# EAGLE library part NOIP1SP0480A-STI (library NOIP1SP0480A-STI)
Image Sensors PYTHON480 1/3.6 BW_ CRA Source: Datasheet
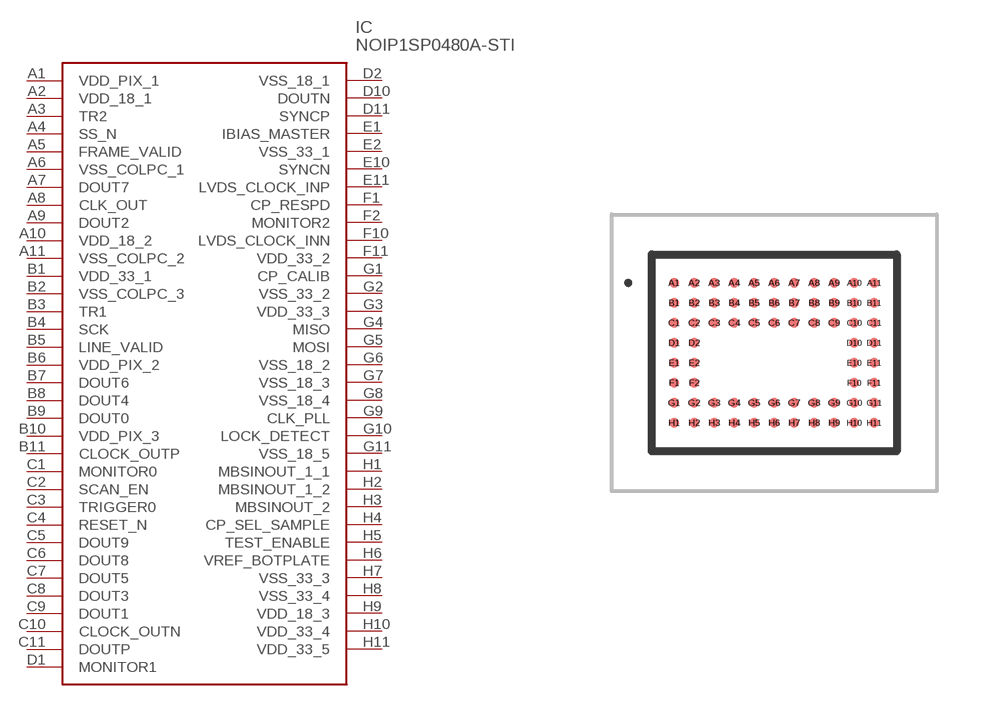
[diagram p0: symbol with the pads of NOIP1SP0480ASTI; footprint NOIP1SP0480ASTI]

Designator prefix IC

## NOIP1SP0480A-STI (Description: Image Sensors PYTHON480 1/3.6 BW_ CRA; Height: 0.75mm; Manufacturer_Name: onsemi; Manufacturer_Part_Number: NOIP1SP0480A-STI; Mouser_Part_Number: 863-NOIP1SP0480A-STI; Mouser_Price-Stock: https://www.mouser.co.uk/ProductDetail/ON-Semiconductor/NOIP1SP0480A-STI?qs=MLItCLRbWsyoZFKf%252BDS9uw%3D%3D)  [NOIP1SP0480ASTI]
A1  VDD_PIX_1
A2  VDD_18_1
A3  TR2
A4  SS_N
A5  FRAME_VALID
A6  VSS_COLPC_1
A7  DOUT7
A8  CLK_OUT
A9  DOUT2
A10  VDD_18_2
A11  VSS_COLPC_2
B1  VDD_33_1
B2  VSS_COLPC_3
B3  TR1
B4  SCK
B5  LINE_VALID
B6  VDD_PIX_2
B7  DOUT6
B8  DOUT4
B9  DOUT0
B10  VDD_PIX_3
B11  CLOCK_OUTP
C1  MONITOR0
C2  SCAN_EN
C3  TRIGGER0
C4  RESET_N
C5  DOUT9
C6  DOUT8
C7  DOUT5
C8  DOUT3
C9  DOUT1
C10  CLOCK_OUTN
C11  DOUTP
D1  MONITOR1
D2  VSS_18_1
D10  DOUTN
D11  SYNCP
E1  IBIAS_MASTER
E2  VSS_33_1
E10  SYNCN
E11  LVDS_CLOCK_INP
F1  CP_RESPD
F2  MONITOR2
F10  LVDS_CLOCK_INN
F11  VDD_33_2
G1  CP_CALIB
G2  VSS_33_2
G3  VDD_33_3
G4  MISO
G5  MOSI
G6  VSS_18_2
G7  VSS_18_3
G8  VSS_18_4
G9  CLK_PLL
G10  LOCK_DETECT
G11  VSS_18_5
H1  MBSINOUT_1_1
H2  MBSINOUT_1_2
H3  MBSINOUT_2
H4  CP_SEL_SAMPLE
H5  TEST_ENABLE
H6  VREF_BOTPLATE
H7  VSS_33_3
H8  VSS_33_4
H9  VDD_18_3
H10  VDD_33_4
H11  VDD_33_5

## Footprint NOIP1SP0480ASTI (pad centres in mm)
NOIP1SP0480A-STI-3
smd 0.25 x 0.25: A1 -2.5,1.75; A2 -2,1.75; A3 -1.5,1.75; A4 -1,1.75; A5 -0.5,1.75; A6 0,1.75; A7 0.5,1.75; A8 1,1.75; A9 1.5,1.75; A10 2,1.75; A11 2.5,1.75; B1 -2.5,1.25; B2 -2,1.25; B3 -1.5,1.25; B4 -1,1.25; B5 -0.5,1.25; B6 0,1.25; B7 0.5,1.25; B8 1,1.25; B9 1.5,1.25; B10 2,1.25; B11 2.5,1.25; C1 -2.5,0.75; C2 -2,0.75; C3 -1.5,0.75; C4 -1,0.75; C5 -0.5,0.75; C6 0,0.75; C7 0.5,0.75; C8 1,0.75; C9 1.5,0.75; C10 2,0.75; C11 2.5,0.75; D1 -2.5,0.25; D2 -2,0.25; D10 2,0.25; D11 2.5,0.25; E1 -2.5,-0.25; E2 -2,-0.25; E10 2,-0.25; E11 2.5,-0.25; F1 -2.5,-0.75; F2 -2,-0.75; F10 2,-0.75; F11 2.5,-0.75; G1 -2.5,-1.25; G2 -2,-1.25; G3 -1.5,-1.25; G4 -1,-1.25; G5 -0.5,-1.25; G6 0,-1.25; G7 0.5,-1.25; G8 1,-1.25; G9 1.5,-1.25; G10 2,-1.25; G11 2.5,-1.25; H1 -2.5,-1.75; H2 -2,-1.75; H3 -1.5,-1.75; H4 -1,-1.75; H5 -0.5,-1.75; H6 0,-1.75; H7 0.5,-1.75; H8 1,-1.75; H9 1.5,-1.75; H10 2,-1.75; H11 2.5,-1.75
